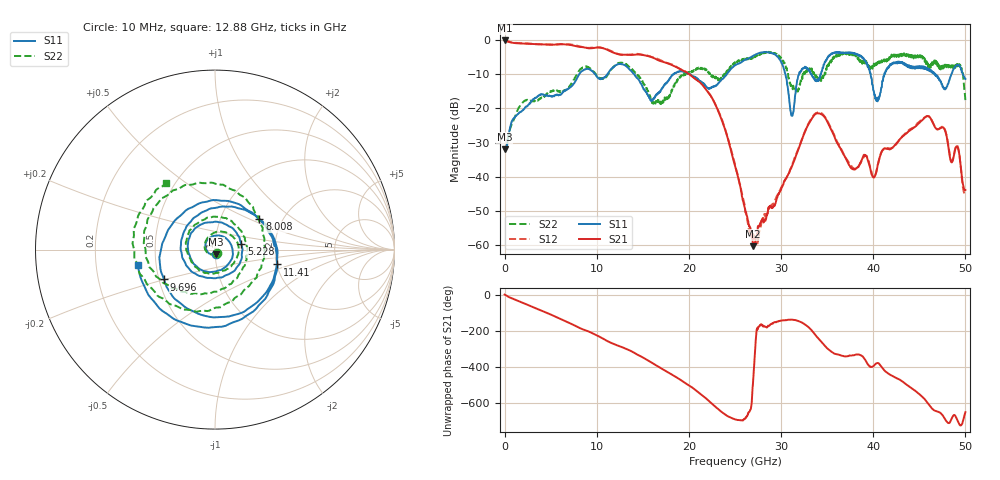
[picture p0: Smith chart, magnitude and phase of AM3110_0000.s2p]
# Hz S DB R 50.0
!freq dBS11 angS11 dBS21 angS21 dBS12 angS12 dBS22 angS22
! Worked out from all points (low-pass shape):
!   1601 points, 10 MHz to 50 GHz, reference 50 ohm
!   highest |S21| = -0.09 dB at 10 MHz (marker M1); lowest = -60.3 dB at 26.97 GHz (marker M2)
!   |S21| within 3 dB of the highest: start of sweep to 11.35 GHz
!   lowest |S11| = -32.0 dB at 10 MHz (marker M3), VSWR 1.05, Z = 50.5 - j2.48 ohm
!   |S11| at or under -10 dB: start of sweep to 8.089 GHz; 14.07 GHz to 18.28 GHz (4.214 GHz wide, 26.1 % of centre); 20.14 GHz to 24.1 GHz (3.962 GHz wide, 17.9 % of centre)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
!   |S22| runs from -32.3 to -3.4 dB; largest |S21 - S12| = 0.023
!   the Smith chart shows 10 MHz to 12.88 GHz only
!   S11 on the Smith chart (normalised r, x): 10 MHz: 1.01, -0.05; 5.228 GHz: 1.34, +0.08; 8.008 GHz: 1.53, +0.58; 9.696 GHz: 0.53, -0.20; 11.41 GHz: 2.02, -0.38; 12.88 GHz: 0.39, -0.08
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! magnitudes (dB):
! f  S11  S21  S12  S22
! 10 MHz  -32.0  -0.1  -0.1  -32.3
! 1.853 GHz  -20.8  -1.0  -0.9  -18.6
! 5.228 GHz  -16.5  -1.3  -1.3  -14.7
! 8.008 GHz  -10.4  -1.9  -1.7  -9.3
! 8.352 GHz  -9.1  -2.0  -1.9  -8.2
! 9.696 GHz  -9.7  -2.3  -2.2  -9.3
! 11.41 GHz  -8.9  -3.2  -3.0  -9.2
! 12.88 GHz  -7.2  -4.3  -4.2  -6.8
! 16.69 GHz  -15.5  -5.9  -5.6  -17.5
! 22.16 GHz  -14.1  -15.5  -15.4  -9.4
! 25 GHz  -7.4  -36.8  -36.5  -6.7
! 26.97 GHz  -4.6  -60.3  -56.8  -4.9
! 29.79 GHz  -5.4  -44.8  -44.4  -4.6
! 31.19 GHz  -22.1  -36.9  -36.5  -13.6
! 32.1 GHz  -9.2  -30.4  -30.2  -12.2
! 33.35 GHz  -10.1  -23.0  -22.7  -8.4
! 37.78 GHz  -3.7  -37.8  -37.4  -3.9
! 40.38 GHz  -17.8  -38.0  -37.9  -7.2
! 41.69 GHz  -7.7  -31.9  -31.7  -5.8
! 46.03 GHz  -8.8  -22.3  -22.3  -7.0
! 49.16 GHz  -7.2  -31.3  -31.1  -7.7
! 50 GHz  -11.3  -43.8  -45.1  -17.6
